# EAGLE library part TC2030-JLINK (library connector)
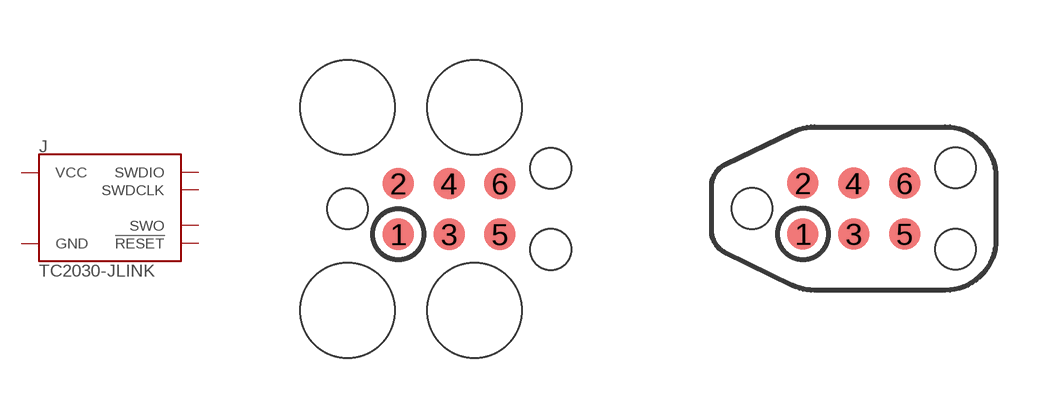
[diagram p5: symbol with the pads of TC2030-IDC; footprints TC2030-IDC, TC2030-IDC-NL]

Designator prefix J

## TC2030-JLINK-L  [TC2030-IDC]
1  VCC
2  SWDIO
3  !RESET
4  SWDCLK
5  GND
6  SWO

## TC2030-JLINK-NL  [TC2030-IDC-NL]
Pads as for TC2030-IDC

## TC2030-JLINK-NL_NOSILK  [TC2030-IDC-NL_NOSILK]
Pads as for TC2030-IDC

## Footprint TC2030-IDC (pad centres in mm)
Tag Connect TC2030-IDC
smd 0.787 x 0.787: 1 -1.27,-0.635; 2 -1.27,0.635; 3 0,-0.635; 4 0,0.635; 5 1.27,-0.635; 6 1.27,0.635
hole 2.375 at -2.54,2.54
hole 2.375 at 0.635,2.54
hole 2.375 at 0.635,-2.54
hole 2.375 at -2.54,-2.54
hole 1.016 at -2.54,0
hole 1.016 at 2.54,1.016
hole 1.016 at 2.54,-1.016

## Footprint TC2030-IDC-NL (pad centres in mm)
The TC2030-IDC-NL is our "No Legs" 6-pin Plug-of-Nails Cable
smd 0.787 x 0.787: 1 -1.27,-0.635; 2 -1.27,0.635; 3 0,-0.635; 4 0,0.635; 5 1.27,-0.635; 6 1.27,0.635
hole 1.016 at -2.54,0
hole 1.016 at 2.54,1.016
hole 1.016 at 2.54,-1.016

## Footprint TC2030-IDC-NL_NOSILK (pad centres in mm)
smd 0.787 x 0.787: 1 -1.27,-0.635; 2 -1.27,0.635; 3 0,-0.635; 4 0,0.635; 5 1.27,-0.635; 6 1.27,0.635
hole 1.016 at -2.54,0
hole 1.016 at 2.54,1.016
hole 1.016 at 2.54,-1.016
